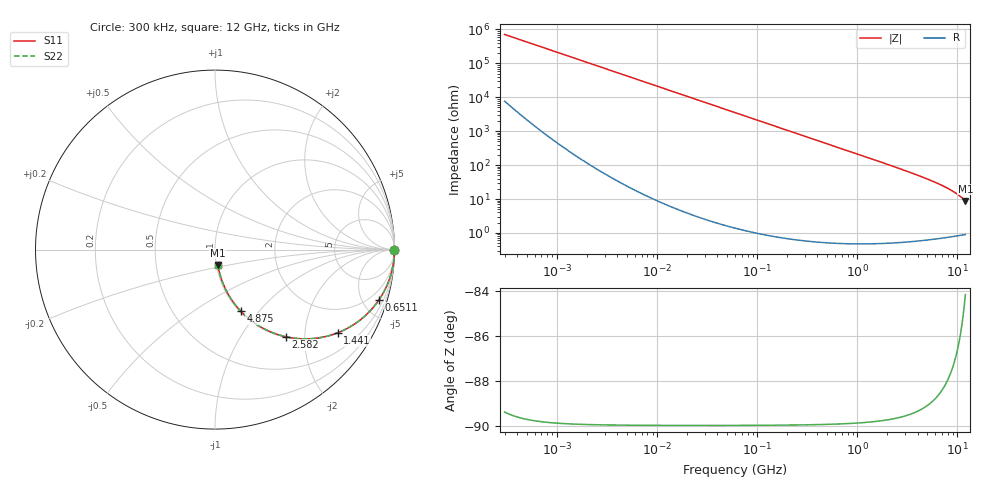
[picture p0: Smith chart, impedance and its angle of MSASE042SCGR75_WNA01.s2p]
! MSASE042SCGR75_WNA01  S-PARAMETER MODEL  ( General Type )
! Model Generated by TAIYO YUDEN Corporation (http://www.ty-top.com)
! Version 1.0
! TAIYO YUDEN Control No. 130801
! Copyright(c) 2013 TAIYO YUDEN CO.,LTD. All Rights Reserved.
! Product Description (link to TY-COMPAS)
! https://ds.yuden.co.jp/TYCOMPAS/or/detail?pn=MSASE042SCGR75AWNA01&u=M
! Products Name : Multilayer Ceramic Capacitors
! Characteristics :
!  Capacitance : 0.75 pF , Rated Voltage : 16V , TCC : CG / C0G
!  Case Size : 0.4 x 0.2 / 0.016 x 0.008 [mm/inch] , Thickness : 0.2 / 0.008 [mm/inch]
!  (Conditions: Temperature = 25 degC , DC Bias Current/Voltage = 0A / 0V)
! External Node Assignments :
!  1  o---| |---o  2
! GND o---------o GND
! Frequency Range : 0.3MHz  -  12000MHz  [ 401 STEP ]
# MHz S RI R 50
! Freq[MHz].  S11 Real  S11 Imag  S21 Real  S21 Imag  S12 Real  S12 Imag  S22 Real  S22 Imag
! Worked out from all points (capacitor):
!   401 points, 300 kHz to 12 GHz, reference 50 ohm
!   read as one part in series: C = 746 fF near 316.3 kHz
!   lowest |Z| = 8.78 ohm at 12 GHz (marker M1)
!   S11 on the Smith chart (normalised r, x): 300 kHz: open; 651.1 MHz: 1.01, -6.54; 1.441 GHz: 1.01, -2.94; 2.582 GHz: 1.01, -1.61; 4.875 GHz: 1.01, -0.80; 12 GHz: 1.02, -0.17
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0.3  1 -0.000141  1.54e-06 0.000141  1.54e-06 0.000141  1 -0.000141
0.316324  1 -0.000148  1.49e-06 0.000148  1.49e-06 0.000148  1 -0.000148
1.769972  1 -0.00083  1.68e-06 0.00083  1.68e-06 0.00083  1 -0.00083
10.44266  1 -0.0049  2.6e-05 0.0049  2.6e-05 0.0049  1 -0.0049
60  0.9992 -0.0281  0.000802 0.0281  0.000802 0.0281  0.9992 -0.0281
164.1901  0.9941 -0.0765  0.00593 0.0765  0.00593 0.0765  0.9941 -0.0765
244.3004  0.987 -0.1131  0.013 0.1131  0.013 0.1131  0.987 -0.1131
353.9943  0.973 -0.1615  0.027 0.1615  0.027 0.1615  0.973 -0.1615
486.4723  0.9502 -0.2168  0.0498 0.2168  0.0498 0.2168  0.9502 -0.2168
651.0506  0.9142 -0.2793  0.0858 0.2793  0.0858 0.2793  0.9142 -0.2793
968.706  0.8275 -0.3767  0.1725 0.3767  0.1725 0.3767  0.8275 -0.3767
1166.079  0.7676 -0.4211  0.2324 0.4211  0.2324 0.4211  0.7676 -0.4211
1441.349  0.6828 -0.4638  0.3172 0.4638  0.3172 0.4638  0.6828 -0.4638
1735.023  0.5963 -0.4886  0.4037 0.4886  0.4037 0.4886  0.5963 -0.4886
2088.533  0.5028 -0.4975  0.4972 0.4975  0.4972 0.4975  0.5028 -0.4975
2581.562  0.3949 -0.4856  0.6051 0.4856  0.6051 0.4856  0.3949 -0.4856
3642.919  0.2397 -0.4219  0.7603 0.4219  0.7603 0.4219  0.2397 -0.4219
4875.354  0.1422 -0.3417  0.8578 0.3417  0.8578 0.3417  0.1422 -0.3417
6524.734  0.077 -0.2546  0.923 0.2546  0.923 0.2546  0.077 -0.2546
8281.503  0.0433 -0.1853  0.9567 0.1853  0.9567 0.1853  0.0433 -0.1853
9708.23  0.0285 -0.1412  0.9715 0.1412  0.9715 0.1412  0.0285 -0.1412
12000  0.0162 -0.0851  0.9838 0.0851  0.9838 0.0851  0.0162 -0.0851
